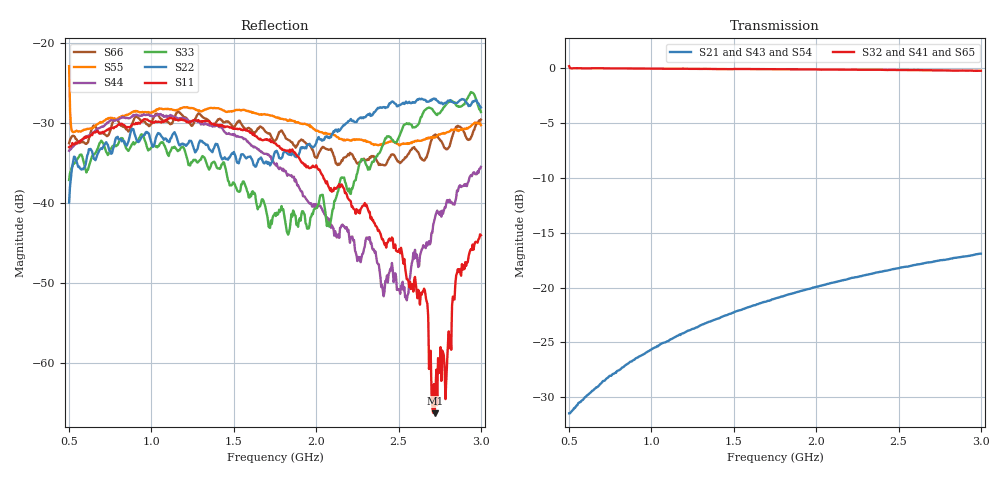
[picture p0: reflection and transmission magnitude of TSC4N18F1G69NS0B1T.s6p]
! TSC4N18F1G69NS0B1T  S-PARAMETER MODEL  ( General Type )
! Model Generated by TAIYO YUDEN Corporation (https://www.yuden.co.jp/en/)
! Version 1.0
! TAIYO YUDEN Control No. 20240527
! Copyright(c) 2024 TAIYO YUDEN CO.,LTD. All Rights Reserved.
! Products Name : Ceramic RF Devices
! Characteristics :
!  Passband freq : 699-2690MHz ( At Passband , Insertion Loss : 0.36dB , Return Loss : 20dB min )
!  Coupling : 17.1dB min 29.5dB max at 699-2690MHz , Directivity : 18dB min 24dB max at 699-2690MHz
!  Case Size : 1.6 x 0.8 / 0.063 x 0.031 [mm/inch] , Thickness : 0.5 / 0.02 [mm/inch]
!  (Conditions: Temperature = 25 degC , DC Bias Current/Voltage = 0A / 0V)
! External Node Assignments :
!  PIN No.8 GND
!  o
! PIN No.1 RF1_IN/OUT(PORT1) o---|-------|---o  PIN No.7 CPL1_RF1(PORT6)
! PIN No.2 CPL2_RF1(PORT2)  o---|  |---o  PIN No.6 CPL1_RF2(PORT5)
! PIN No.3 CPL2_RF2(PORT3)  o---|-------|---o  PIN No.5 RF2_OUT/IN(PORT4)
!  o
!  PIN No.4 GND
! Frequency Range : 500MHz  -  3GHz  [ 2501 STEP ]
# MHz S RI R 50
! Freq[MHz].  S11 Real  S11 Imag  S12 Real  S12 Imag  S13 Real  S13 Imag  S14 Real  S14 Imag
!  S15 Real  S15 Imag  S16 Real  S16 Imag
!  S21 Real  S21 Imag  S22 Real  S22 Imag  S23 Real  S23 Imag  S24 Real  S24 Imag
!  S25 Real  S25 Imag  S26 Real  S26 Imag
!  S31 Real  S31 Imag  S32 Real  S32 Imag  S33 Real  S33 Imag  S34 Real  S34 Imag
!  S35 Real  S35 Imag  S36 Real  S36 Imag
!  S41 Real  S41 Imag  S42 Real  S42 Imag  S43 Real  S43 Imag  S44 Real  S44 Imag
!  S45 Real  S45 Imag  S46 Real  S46 Imag
!  S51 Real  S51 Imag  S52 Real  S52 Imag  S53 Real  S53 Imag  S54 Real  S54 Imag
!  S55 Real  S55 Imag  S56 Real  S56 Imag
!  S61 Real  S61 Imag  S62 Real  S62 Imag  S63 Real  S63 Imag  S64 Real  S64 Imag
!  S65 Real  S65 Imag  S66 Real  S66 Imag
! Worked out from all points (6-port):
!   2501 points, 500 MHz to 3 GHz, reference 50 ohm
!   strongest paths, dB at 500 MHz, 1.125 GHz, 1.75 GHz, 2.375 GHz, 3 GHz:
!     S32: 0.2, 0.0, -0.1, -0.1, -0.2
!     S41: 0.0, 0.0, -0.1, -0.2, -0.3
!     S65: 0.5, -0.1, -0.1, -0.2, -0.2
!     S21: -31.5, -24.7, -21.0, -18.6, -16.9
!     S43: -31.5, -24.7, -21.0, -18.6, -16.9
!     S54: -31.6, -24.7, -21.0, -18.6, -17.0
!   lowest |S11| = -66.3 dB at 2.72 GHz (marker M1), VSWR 1.00, Z = 50 + j0.00137 ohm
!   |S11| at or under -10 dB: start of sweep to end of sweep
